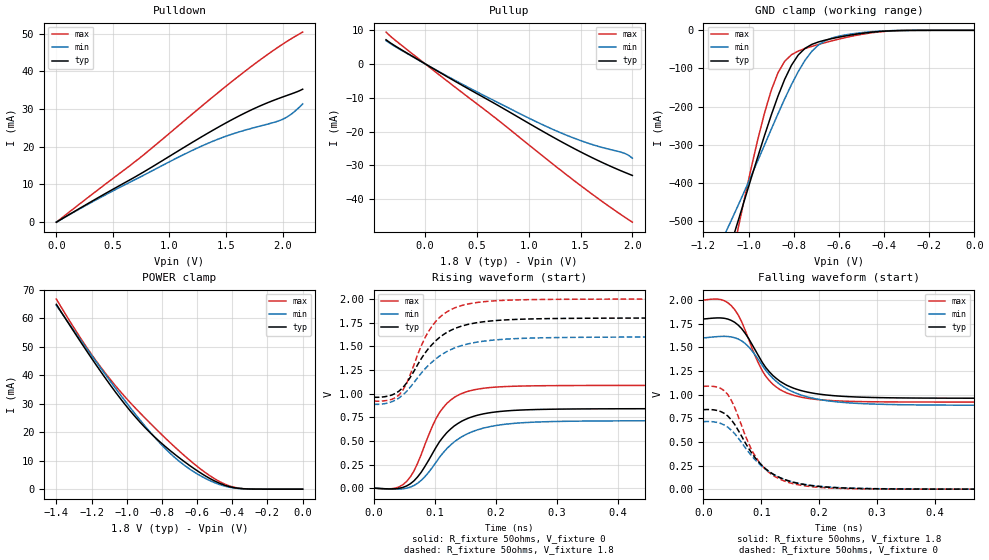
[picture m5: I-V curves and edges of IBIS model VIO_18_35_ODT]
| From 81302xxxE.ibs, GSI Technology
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|  signals   DQA1-DQA9, DQB1-DQB9, DQC1-DQC9, DQD1-DQD9
[Model]   VIO_18_35_ODT
Model_type   I/O
Polarity   Non-Inverting
Vinl  =   0.7000V
Vinh  =   1.1000V
Vmeas =   0.90v
Rref  =   50
|  variable   typ   min   max
C_comp   3.0pF   2.5pF   3.5pF
[Receiver Thresholds]
Vth = 0.90V
Vth_min = 0.80V
Vth_max = 0.95V
Threshold_sensitivity = 1.0
Reference_supply Ext_ref
Vinh_ac = +200mv
Vinh_dc = +100mv
Vinl_ac = -200mv
Vinl_dc = -100mv
Tslew_ac = 550ps
|  variable   typ   min   max
[External Reference]   0.90   0.80   0.95
|  variable   typ   min   max
[Temperature Range]   50   100   0
|  variable   typ   min   max
[Voltage Range]   1.8   1.6   2.0
[Add Submodel]
| Submodel Name   Mode
Weak_ODT_15V   Non-Driving
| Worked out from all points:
|   slope of the pulldown table from 0 to 0.27 V, typ, clamps not added: 56.5 ohm
|   slope of the pullup table from 0 to 0.27 V, typ, clamps not added: 56.1 ohm
|   GND clamp passes 1 mA (typ) near -0.36 V on its own axis
|   POWER clamp passes 1 mA (typ) near -0.42 V on its own axis
|   rising waveform, R_fixture 50ohms, V_fixture 0: 20-80 % time 57.5ps typ, 65.6ps min, 47.7ps max; typ from 0 V to 0.841 V
|   rising waveform, R_fixture 50ohms, V_fixture 1.8: 20-80 % time 60.6ps typ, 69ps min, 49ps max; typ from 0.962 V to 1.8 V
|   falling waveform, R_fixture 50ohms, V_fixture 1.8: 20-80 % time 61.5ps typ, 69.7ps min, 50.7ps max; typ from 1.8 V to 0.962 V
|   falling waveform, R_fixture 50ohms, V_fixture 0: 20-80 % time 62.9ps typ, 69.1ps min, 52.3ps max; typ from 0.841 V to 0 V
[Pullup]
| V(VDDQ-Vout)   typ   min   max
-376mV    7.091mA    6.812mA    9.353mA
-256mV    4.665mA    4.498mA    6.17mA
296mV     -5.271mA   -4.998mA   -7.043mA
680mV     -11.87mA   -11.08mA   -16.03mA
1.088V    -19.1mA    -17.32mA   -26.07mA
1.328V    -23.22mA   -20.61mA   -31.88mA
1.568V    -27.05mA   -23.38mA   -37.48mA
1.904V    -31.76mA   -26.21mA   -44.8mA
1.952V    -32.36mA   -26.82mA   -45.79mA
2V        -32.95mA   -27.87mA   -46.75mA
[PullDown]
| voltage   typ   min   max
0V        -6.816nA   -13.22nA   -7.579nA
352mV     6.199mA    5.933mA    8.214mA
704mV     12.14mA    11.41mA    16.24mA
1.056V    18.5mA     16.88mA    24.99mA
1.32V     23.27mA    20.65mA    31.64mA
1.518V    26.63mA    22.99mA    36.48mA
1.76V     30.28mA    25.16mA    42.12mA
1.98V     32.97mA    27.03mA    46.79mA
2.068V    33.92mA    28.46mA    48.48mA
2.178V    35.27mA    31.38mA    50.42mA
[POWER Clamp]
|V(VDDQ-Vout)   typ   min   max
-1.4V     64.83mA    64.49mA    66.68mA
-1.288V   54.1mA     54.59mA    55.43mA
-1.176V   43.77mA    44.87mA    45.19mA
-1.092V   36.42mA    37.75mA    38.39mA
-980mV    27.45mA    28.59mA    30.36mA
-896mV    21.62mA    22.13mA    24.95mA
-812mV    16.64mA    16.22mA    19.79mA
-672mV    9.628mA    8.359mA    11.74mA
-504mV    2.977mA    2.36mA     3.78mA
-392mV    542uA      426.3uA    698.9uA
-308mV    66uA       60.25uA    73.63uA
0V        32.31nA    56.32nA    14.02nA
[GND Clamp]
|(Vout)   typ   min   max
-1.5V     -1.259A    -998.1mA   -1.702A
-1.11V    -621.1mA   -540.5mA   -701.3mA
-1.08V    -564.5mA   -502.7mA   -615.1mA
-1.05V    -506.9mA   -463.9mA   -529.8mA
-930mV    -276.8mA   -301.4mA   -218.1mA
-900mV    -223mA     -260.1mA   -157.9mA
-870mV    -172.8mA   -219.3mA   -111.5mA
-810mV    -91.53mA   -142.2mA   -64mA
-720mV    -36.92mA   -55.09mA   -42.15mA
-630mV    -21.52mA   -20.02mA   -27.43mA
-390mV    -1.864mA   -1.3mA     -2.486mA
0V        -8.791nA   -16.65nA   -9.225nA
[Ramp]
| voltage   typ   min   max
dV/dt_r   0.54/186p   0.48/213p   0.60/209p
dV/dt_f   0.86/129p   0.66/166p   1.07/101p
R_load  =   50ohms
[Rising Waveform]
R_fixture =   50ohms
V_fixture =   0
| Time   V(typ)   V(min)   V(max)
0s        179.6nV    353.4nV    173.7nV
36ps      -6.036mV   -10.67mV   1.673mV
54ps      23.57mV    -42.3uV    71.33mV
66ps      77.73mV    28.06mV    182.7mV
78ps      170.1mV    83.41mV    358.3mV
108ps     493.1mV    328.3mV    801.9mV
132ps     658.4mV    490.1mV    960.7mV
156ps     742.9mV    582.6mV    1.027V
258ps     830.1mV    696.7mV    1.082V
600ps     840.8mV    713.6mV    1.087V
[Rising Waveform]
R_fixture =   50ohms
V_fixture =   1.8
V_fixture_min =  1.6
V_fixture_max =  2.0
| Time   V(tyn)   V(min)   V(max)
0s        961.7mV    887.1mV    921.1mV
24ps      974.4mV    902.1mV    929.8mV
42ps      1.029V     956.3mV    989.2mV
54ps      1.113V     1.024V     1.11V
78ps      1.371V     1.217V     1.506V
96ps      1.522V     1.336V     1.717V
120ps     1.648V     1.446V     1.865V
144ps     1.714V     1.508V     1.932V
252ps     1.789V     1.586V     1.994V
600ps     1.8V       1.6V       2V
[Falling Waveform]
R_fixture =   50ohms
V_fixture =   1.8
V_fixture_min = 1.6
V_fixture_max = 2.0
| Time   V(typ)   V(min)   V(max)
0s        1.8V       1.6V       2V
30ps      1.811V     1.616V     2.006V
48ps      1.785V     1.61V      1.942V
60ps      1.736V     1.588V     1.843V
78ps      1.594V     1.506V     1.589V
108ps     1.284V     1.254V     1.191V
132ps     1.142V     1.109V     1.054V
156ps     1.067V     1.025V     992.1mV
270ps     973.7mV    906.1mV    926.6mV
600ps     961.7mV    887.2mV    921.1mV
[Falling Waveform]
R_fixture =   50ohms
V_fixture =   0
| Time   V(typ)   V(min)   V(max)
0s        841mV      713.9mV    1.087V
24ps      832.2mV    705.5mV    1.08V
42ps      774.2mV    655.5mV    1.002V
54ps      684.8mV    586.9mV    865.4mV
84ps      376.4mV    346.8mV    404.2mV
96ps      284.5mV    270.4mV    286.9mV
120ps     160.3mV    159.2mV    146.6mV
144ps     92.74mV    95.19mV    76.73mV
252ps     10.17mV    12.05mV    5.692mV
600ps     27.4uV     68.12uV    5.325uV
